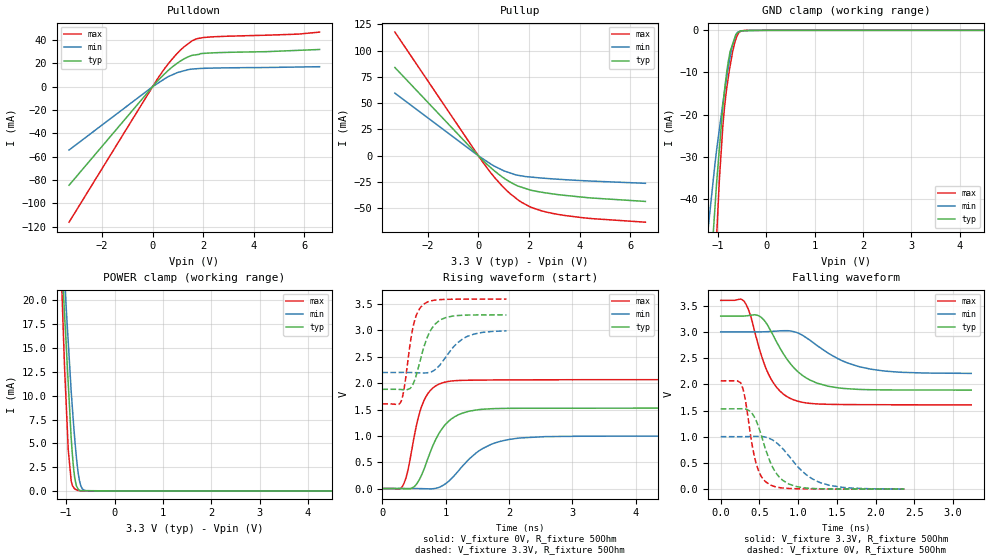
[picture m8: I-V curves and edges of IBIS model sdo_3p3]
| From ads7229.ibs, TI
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|   sdo_3p3 Model
[Model]   sdo_3p3
Model_type   3-state
Polarity   Non-Inverting
Vmeas = 1.65
Vref = 1.65
Cref = 30pF
Rref = 50
|   typ   min   max
|   (nom PVT)   (Fast PVT)   (slow PVT)
|C_comp from frequency sweep method(F=50MHz)
C_comp   5.061e-12   4.100e-12   5.975e-12
|OFF state: BUFFER IN HIGH IMPEDANCE
|C_comp   5.061e-12   4.100e-12   5.975e-12
|ON state : BUFFER OUTPUT TURNED HIGH
|C_comp   5.474e-12   4.490e-12   6.450e-12
|C_comp from LC tank measurement(L=1nH)
|ON state : BUFFER OUTPUT TURNED HIGH
|Resonant Frequency(Hz)   2.450e+09   2.630e+09   2.340e+09
|C_comp   4.224e-12   3.666e-12   4.631e-12
|OFF state: BUFFER IN HIGH IMPEDANCE
|Resonant Frequency   2.550e+09   2.800e+09   2.390e+09
|C_comp   3.899e-12   3.234e-12   4.439e-12
| Where nom  PVT is Nominal Process,  3.3V,  28C
|   Fast PVT is Strong Process,   3.6V,  -40C
|   Slow PVT is Weak Process,   3V,  88C
[Voltage Range]   3.3   3   3.6
|Ambient Temperature   25   85   -40
|Junction Temperature
[Temperature Range]   28   88   -40
[Pullup Reference]   3.3   3   3.6
[Pulldown Reference]   0   0   0
[Power Clamp Reference]   3.3   3   3.6
[GND Clamp Reference]   0   0   0
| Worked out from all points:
|   slope of the pulldown table from 0 to 0.495 V, typ, clamps not added: 43.3 ohm
|   slope of the pullup table from 0 to 0.495 V, typ, clamps not added: 43.4 ohm
|   GND clamp passes 1 mA (typ) near -0.62 V on its own axis
|   POWER clamp passes 1 mA (typ) near -0.81 V on its own axis
|   falling waveform, V_fixture 3.3V, R_fixture 50Ohm: 20-80 % time 408ps typ, 570ps min, 285ps max; typ from 3.3 V to 1.89 V
|   rising waveform, V_fixture 0V, R_fixture 50Ohm: 20-80 % time 367ps typ, 553ps min, 238ps max; typ from 0 V to 1.53 V
|   rising waveform, V_fixture 3.3V, R_fixture 50Ohm: 20-80 % time 228ps typ, 342ps min, 154ps max; typ from 1.88 V to 3.29 V
|   falling waveform, V_fixture 0V, R_fixture 50Ohm: 20-80 % time 236ps typ, 396ps min, 150ps max; typ from 1.53 V to 0.008 V
[Pulldown]
|   Voltage   I(typ)   I(min)   I(max)
-3.3V     -84.5mA    -54.28mA   -116.2mA
172.8mV   4.321mA    2.494mA    5.996mA
648mV     14.59mA    8.972mA    20.48mA
939.6mV   19.67mA    11.76mA    27.86mA
1.246V    23.91mA    13.75mA    34.31mA
1.57V     26.96mA    15.2mA     39.49mA
1.811V    27.73mA    15.59mA    41.49mA
2.012V    28.63mA    15.79mA    42.21mA
5.774V    31.25mA    16.94mA    45.18mA
6.6V      31.99mA    17.21mA    46.91mA
[GND Clamp]
|   Voltage   I(typ)   I(min)   I(max)
-3.3V     -515.1mA   -360.9mA   -728.9mA
-1.236V   -72.97mA   -50.81mA   -106.6mA
-1.185V   -63.28mA   -45.24mA   -92.2mA
-1.059V   -41.88mA   -31.6mA    -56.9mA
-1.023V   -35.76mA   -28.13mA   -48.27mA
-896.4mV  -18.01mA   -17.25mA   -22.62mA
-820.8mV  -10.27mA   -11.41mA   -14.07mA
-745.8mV  -5.02mA    -6.286mA   -8.385mA
-696mV    -3.367mA   -3.336mA   -5.168mA
-612mV    -861uA     -747uA     -1.512mA
-537mV    -199uA     -155.1uA   -329.7uA
6.6V      0A         0A         0A
[Pullup]
|   Voltage   I(typ)   I(min)   I(max)
-3.3V     83.87mA    59.52mA    117.5mA
172.8mV   -4.243mA   -2.787mA   -6.008mA
583.2mV   -13.3mA    -9.192mA   -18.99mA
939.6mV   -20.06mA   -13.5mA    -28.71mA
1.246V    -24.85mA   -16.26mA   -35.81mA
1.588V    -28.94mA   -18.64mA   -42.32mA
2.167V    -33.2mA    -20.45mA   -49.72mA
3.089V    -36.75mA   -22.21mA   -55.5mA
4.496V    -40.17mA   -24.1mA    -59.74mA
6.6V      -43.38mA   -26.18mA   -63.12mA
[POWER Clamp]
|   Voltage   I(typ)   I(min)   I(max)
-3.3V     177.2mA    159.9mA    202.3mA
-1.451V   64.21mA    57.65mA    74.34mA
-1.053V   20.33mA    23.74mA    15.72mA
-1.033V   18.48mA    22.08mA    12.9mA
-957.6mV  11.31mA    15.64mA    4.341mA
-896.4mV  5.542mA    10.44mA    1.014mA
-858mV    2.968mA    7.716mA    450.9uA
-825mV    1.431mA    5.571mA    220.1uA
-756mV    227.7uA    2.041mA    37.91uA
-696mV    34.33uA    508.2uA    6.822uA
-591mV    29.13uA    21.79uA    1.713uA
6.6V      0A         0A         0A
[Ramp]
R_load = 50
|   typ   min   max
dV/dt_r   0.919499/3.66106e-10   0.600271/5.474e-10   1.24222/2.37161e-10
dV/dt_f   0.848902/4.11862e-10   0.476909/5.71963e-10   1.19684/2.85358e-10
[Falling Waveform]
V_fixture = 3.3V
V_fixture_min = 3V
V_fixture_max = 3.6V
R_fixture = 50Ohm
|   Time   V(typ)   V(min)   V(max)
0s        3.3V       3V         3.6V
303ps     3.302V     3V         3.579V
384ps     3.316V     3V         3.314V
486ps     3.31V      3V         2.744V
610ps     3.117V     3.005V     2.219V
756ps     2.717V     3.019V     1.887V
927ps     2.347V     3.01V      1.715V
1.257ns   2.019V     2.727V     1.627V
1.81ns    1.904V     2.33V      1.615V
3.236ns   1.892V     2.21V      1.61V
[Rising Waveform]
V_fixture = 0V
V_fixture_min = 0V
V_fixture_max = 0V
R_fixture = 50Ohm
|   Time   V(typ)   V(min)   V(max)
0s        1.151nV    1.335nV    1.032nV
319ps     -1.204mV   235.7uV    44.64mV
403ps     -6.918mV   405.5uV    342.1mV
505ps     36.81mV    207.9uV    1.001V
604ps     216.1mV    -1.343mV   1.5V
713ps     552.4mV    -5.187mV   1.792V
1.051ns   1.282V     142.3mV    2.034V
1.58ns    1.504V     756.8mV    2.059V
2.198ns   1.523V     961.5mV    2.063V
10ns      1.532V     1V         2.07V
[Rising Waveform]
V_fixture = 3.3V
V_fixture_min = 3V
V_fixture_max = 3.6V
R_fixture = 50Ohm
|   Time   V(typ)   V(min)   V(max)
0s        1.883V     2.203V     1.605V
296ps     1.879V     2.203V     1.654V
355ps     1.874V     2.203V     1.98V
488ps     1.992V     2.201V     3.082V
546ps     2.195V     2.198V     3.318V
637ps     2.611V     2.193V     3.482V
767ps     3.013V     2.21V      3.562V
936ps     3.213V     2.386V     3.587V
1.326ns   3.292V     2.879V     3.595V
1.96ns    3.295V     2.992V     3.596V
[Falling Waveform]
V_fixture = 0V
V_fixture_min = 0V
V_fixture_max = 0V
R_fixture = 50Ohm
|   Time   V(typ)   V(min)   V(max)
0s        1.534V     1.005V     2.068V
260ps     1.537V     1.005V     2.024V
314ps     1.532V     1.006V     1.739V
455ps     1.319V     1.011V     508.4mV
525ps     1.029V     1.007V     244.8mV
623ps     584.5mV    974.7mV    101.3mV
730ps     282.4mV    878.1mV    42.98mV
882ps     102.3mV    635.8mV    18.82mV
1.284ns   13.56mV    131mV      9.029mV
2.373ns   8.048mV    7.4mV      5.55mV
